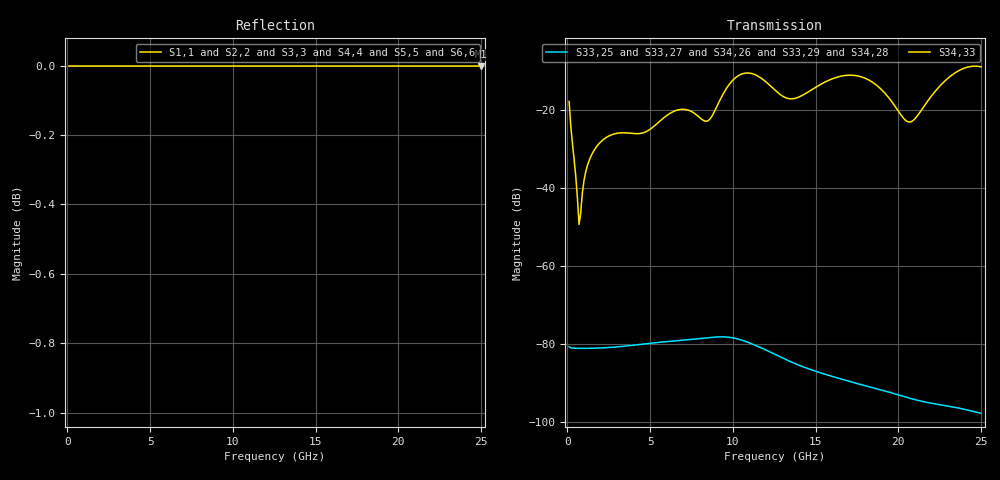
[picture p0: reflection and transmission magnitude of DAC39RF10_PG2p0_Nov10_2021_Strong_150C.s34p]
! Touchstone Ver. 1.0
! Number of ports is 34
# Hz	S	RI	R	50.000000
! SCATTERING PARAMETERS  :
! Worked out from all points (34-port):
!   250 points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, 100 MHz to 25 GHz, reference 50 ohm
!   strongest paths, dB at 100 MHz, 6.3 GHz, 12.6 GHz, 18.8 GHz, 25 GHz:
!     S34,33: -17.7, -20.6, -15.0, -14.0, -8.9
!     S33,25: -80.7, -79.3, -82.7, -91.6, -97.8
!     S33,27: -80.7, -79.3, -82.8, -91.6, -97.9
!     S34,26: -80.7, -79.3, -82.8, -91.6, -97.8
!     S33,29: -80.7, -79.3, -82.8, -91.7, -97.9
!     S34,28: -80.7, -79.3, -82.8, -91.6, -97.9
!   lowest |S11| = 0.0 dB at 25 GHz (marker M1)
!   |S11| at or under -10 dB: nowhere
